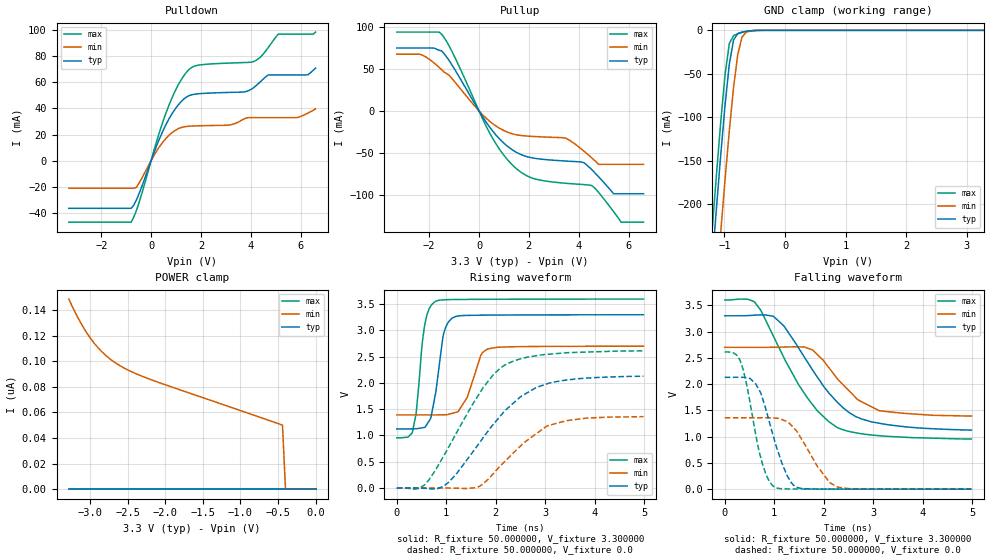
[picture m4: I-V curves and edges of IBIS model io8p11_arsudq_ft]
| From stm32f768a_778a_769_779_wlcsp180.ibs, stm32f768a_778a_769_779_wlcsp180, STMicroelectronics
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|   Model io8p11_arsudq_ft
[Model]  io8p11_arsudq_ft
Model_type I/O
Polarity   Non-Inverting
Enable   Active-Low
Vinl =   0.990000V
Vinh =   2.310000V
Vmeas =  1.650000V
Cref =   30.000000pF
Rref =   100.000000M
Vref =   0.0V
C_comp   2.292100pF   2.228000pF   2.366600pF
[Temperature Range]   25.000000   0.125000k   -40.000000
[Pullup Reference]   3.300000V   2.700000V   3.600000V
[Pulldown Reference]   0.0V   0.0V   0.0V
[POWER Clamp Reference]   3.300000V   2.700000V   3.600000V
[GND Clamp Reference]   0.0V   0.0V   0.0V
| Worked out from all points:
|   slope of the pulldown table from 0 to 0.495 V, typ, clamps not added: 20.9 ohm
|   slope of the pullup table from 0 to 0.495 V, typ, clamps not added: 22.6 ohm
|   GND clamp passes 1 mA (typ) near -0.62 V on its own axis
|   rising waveform, R_fixture 50.000000, V_fixture 3.300000: 20-80 % time 197ps typ, 293ps min, 161ps max; typ from 1.12 V to 3.3 V
|   rising waveform, R_fixture 50.000000, V_fixture 0.0: 20-80 % time 1.13ns typ, 947ps min, 999ps max; typ from 0 V to 2.13 V
|   falling waveform, R_fixture 50.000000, V_fixture 3.300000: 20-80 % time 1.01ns typ, 786ps min, 979ps max; typ from 3.3 V to 1.12 V
|   falling waveform, R_fixture 50.000000, V_fixture 0.0: 20-80 % time 415ps typ, 536ps min, 332ps max; typ from 2.13 V to 0 V
[Pulldown]
|Voltage   I(typ)   I(min)   I(max)
-3.3V     -36.46mA   -21.09mA   -47.09mA
-800mV    -36.46mA   -21.09mA   -47.09mA
-600mV    -30.5mA    -20.54mA   -38.69mA
700mV     31.4mA     19.11mA    41.71mA
1.2V      45.15mA    25.37mA    61.75mA
1.6V      50.35mA    26.5mA     71.06mA
3.1V      52.28mA    27.26mA    74.76mA
4.1V      55.7mA     33mA       75.81mA
4.7V      65.72mA    33mA       86.7mA
5.1V      65.72mA    33mA       96.91mA
6.3V      65.88mA    36.51mA    96.91mA
6.6V      70.94mA    39.72mA    98.51mA
[Pullup]
|Voltage   I(typ)   I(min)   I(max)
-3.3V     74.74mA    67.41mA    93.65mA
-2.3V     74.74mA    66.57mA    93.65mA
-1.5V     71.37mA    49mA       91.08mA
500mV     -22.07mA   -14mA      -30.03mA
1.6V      -50.64mA   -28.81mA   -70.96mA
3.5V      -59.53mA   -32.65mA   -85.92mA
4.2V      -61.43mA   -47.49mA   -87.46mA
4.5V      -69.07mA   -55.12mA   -88.38mA
4.8V      -78.22mA   -63.4mA    -96.83mA
5.4V      -98.3mA    -63.4mA    -119.6mA
5.7V      -98.3mA    -63.4mA    -132.1mA
6.6V      -98.3mA    -63.4mA    -132.1mA
[GND_clamp]
|Voltage   I(typ)   I(min)   I(max)
-3.3V     -2.316A    -2.396A    -2.289A
-1.2V     -265.5mA   -356.1mA   -227.2mA
-1.13V    -202.6mA   -292.9mA   -164.1mA
-1.06V    -142.2mA   -231.2mA   -104.1mA
-990mV    -85.98mA   -171.6mA   -50.72mA
-920mV    -38.8mA    -115.5mA   -15.28mA
-850mV    -11.08mA   -65.6mA    -6.001mA
-780mV    -3.782mA   -27.42mA   -3.876mA
-710mV    -2.086mA   -7.69mA    -2.381mA
-640mV    -1.147mA   -2.118mA   -1.22mA
-570mV    -523.9uA   -798.4uA   -476.8uA
3.28V     0A         0A         0A
[POWER_clamp]
|Voltage   I(typ)   I(min)   I(max)
-3.28V    0A         148.5nA    0A
-3.2V     0A         138.6nA    0A
-3.12V    0A         129.7nA    0A
-3.04V    0A         122nA      0A
-2.96V    0A         115.3nA    0A
-2.8V     0A         105.1nA    0A
-2.6V     0A         96.44nA    0A
-2.4V     0A         90.52nA    0A
-2.16V    0A         84.97nA    0A
-440mV    0A         50.04nA    0A
-400mV    0A         0A         0A
0V        0A         0A         0A
[Ramp]
| variable   typ   min   max
dV/dt_r  1.26126/1.11615n   0.80556/0.93867n   1.56060/0.99645n
dV/dt_f  1.27686/0.99477n   0.77076/0.76219n   1.56992/0.97160n
R_load = 50.000000
[Rising Waveform]
R_fixture= 50.000000
V_fixture= 3.300000
V_fixture_min= 2.700000
V_fixture_max= 3.600000
|time   V(typ)   V(min)   V(max)
0s        1.124V     1.392V     954.3mV
320.3ps   1.126V     1.392V     1.079V
390.4ps   1.128V     1.392V     1.414V
560.6ps   1.153V     1.392V     3.085V
690.7ps   1.345V     1.391V     3.473V
780.8ps   1.788V     1.391V     3.553V
951ps     2.954V     1.395V     3.585V
1.171ns   3.26V      1.435V     3.59V
1.842ns   3.293V     2.649V     3.595V
4.985ns   3.3V       2.7V       3.599V
[Rising Waveform]
R_fixture= 50.000000
V_fixture= 0.0
V_fixture_min= 0.0
V_fixture_max= 0.0
|time   V(typ)   V(min)   V(max)
0s        345.6uV    196.9uV    652.1uV
470.5ps   -2.823mV   136.3uV    -128.9uV
650.7ps   -14.08mV   197.4uV    155.2mV
951ps     37.14mV    -1.041mV   616.4mV
1.662ns   848.1mV    26.71mV    1.787V
2.182ns   1.469V     504.3mV    2.341V
2.503ns   1.739V     801.6mV    2.461V
3.043ns   1.986V     1.184V     2.546V
3.854ns   2.094V     1.333V     2.59V
4.985ns   2.129V     1.359V     2.612V
[Falling Waveform]
R_fixture= 50.000000
V_fixture= 3.300000
V_fixture_min= 2.700000
V_fixture_max= 3.600000
|time   V(typ)   V(min)   V(max)
0s        3.3V       2.7V       3.599V
600.6ps   3.312V     2.7V       3.567V
740.7ps   3.316V     2.7V       3.385V
981ps     3.291V     2.701V     2.918V
1.201ns   3.101V     2.705V     2.493V
1.772ns   2.274V     2.651V     1.614V
2.272ns   1.658V     2.105V     1.173V
2.693ns   1.365V     1.7V       1.066V
3.123ns   1.254V     1.493V     1.018V
4.985ns   1.124V     1.392V     954.3mV
[Falling Waveform]
R_fixture= 50.000000
V_fixture= 0.0
V_fixture_min= 0.0
V_fixture_max= 0.0
|time   V(typ)   V(min)   V(max)
0s        2.129V     1.359V     2.612V
310.3ps   2.129V     1.358V     2.454V
450.5ps   2.118V     1.358V     1.961V
720.7ps   1.845V     1.359V     627.5mV
880.9ps   1.352V     1.359V     186mV
1.011ns   914.8mV    1.352V     40.06mV
1.391ns   74.02mV    1.169V     3.516mV
1.872ns   3.692mV    435.7mV    2.251mV
2.282ns   2.046mV    39.84mV    1.82mV
4.985ns   345.6uV    196.9uV    652.1uV
